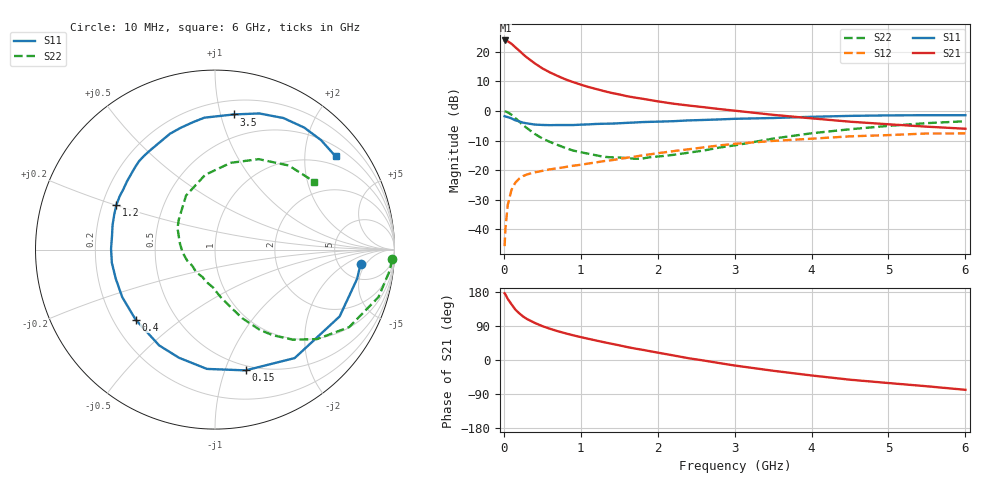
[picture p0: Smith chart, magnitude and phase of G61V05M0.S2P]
! SIEMENS Small Signal Semiconductors
! BFG193
! Si NPN RF Bipolar Junction Transistor in SOT223
! VCE = 1 V  IC = 5 mA
! Common Emitter S-Parameters:  August  1996
# GHz  S  MA  R  50
!  f  S11  S21  S12  S22
! GHz  MAG  ANG  MAG  ANG  MAG  ANG  MAG  ANG
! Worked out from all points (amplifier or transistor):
!   36 points, 10 MHz to 6 GHz, reference 50 ohm
!   highest |S21| = 23.8 dB at 20 MHz (marker M1)
!   |S21| within 3 dB of that: start of sweep to 180.4 MHz
!   unconditionally stable (mu >= 1): 1.06 GHz to 2.934 GHz
!   at 250 MHz: K = 0.35, MSG = 20.6 dB, |S12| = -22.0 dB
!   at 1.4 GHz: K = 1.11, MAG = 9.4 dB, |S12| = -16.6 dB
!   at 6 GHz: K = 0.97, MSG = 0.8 dB, |S12| = -7.6 dB
!   S11 on the Smith chart (normalised r, x): 10 MHz: 7.88, -3.87; 150 MHz: 0.45, -1.18; 400 MHz: 0.29, -0.35; 1.2 GHz: 0.26, +0.20; 3.5 GHz: 0.31, +1.10; 6 GHz: 0.74, +2.75
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0.01  0.8149 -5.8  15.52 176.1  0.0052 88.0  0.9868 -3.2
0.02  0.8083 -11.6  15.54 173.3  0.0101 83.8  0.9818 -6.6
0.05  0.788 -28.2  15.06 161.4  0.0256 74.6  0.9487 -16.2
0.1  0.7499 -53.7  13.65 146.9  0.0467 64.6  0.8634 -30.0
0.15  0.6941 -75.8  11.9 132.9  0.0616 53.8  0.7559 -41.3
0.2  0.6663 -93.9  10.46 123.3  0.0718 47.8  0.6631 -49.2
0.25  0.6352 -108.4  9.087 114.9  0.0795 42.8  0.5765 -55.9
0.3  0.6179 -120.2  8.01 108.2  0.0846 39.6  0.5141 -60.7
0.4  0.5899 -138.6  6.405 98.1  0.0918 35.7  0.4117 -68.3
0.5  0.5807 -152.9  5.25 89.4  0.0973 33.4  0.3432 -73.7
0.6  0.5762 -163.8  4.481 82.4  0.1033 32.6  0.2997 -78.3
0.7  0.5794 -172.8  3.901 76.1  0.1078 32.2  0.2664 -83.2
0.9  0.5786 172.8  3.078 65.3  0.1187 32.0  0.2147 -92.0
1.1  0.5941 161.0  2.544 55.9  0.1294 32.0  0.1894 -103.0
1.2  0.6035 155.6  2.352 51.4  0.1354 31.9  0.1784 -108.6
1.6  0.6298 137.6  1.778 34.3  0.1625 29.8  0.1601 -134.5
2.2  0.6721 117.4  1.33 12.2  0.2094 23.2  0.1811 -175.0
2.8  0.7202 99.9  1.079 -8.1  0.2619 13.2  0.2408 150.1
3.5  0.7605 82.0  0.861 -28.4  0.312 -2.2  0.3414 118.2
4.5  0.8263 62.5  0.659 -52.0  0.3728 -21.5  0.4914 79.7
5.5  0.8492 45.9  0.543 -69.3  0.4165 -45.0  0.6235 48.7
6  0.8492 37.7  0.501 -78.7  0.4176 -58.4  0.67 34.3
